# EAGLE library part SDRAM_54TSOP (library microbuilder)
64Mb SDRAM (4Mb x 16) Micron: MT48LC4M16A2P-7E:G TR - 133 MHz, 3V-3.6V, 0-70C - Digikey: 557-1089-1-ND MT48LC4M16A2P-75 IT:G TR - 133 MHz, 3V-3.6V, -40-85C - Digikey: 557-1087-1-ND ISSI (cheaper): IS42S16400F-7TL - 143 MHz, 3V-3.6V, 0-70C - Digikey: 706-1077-ND IS42S16400J-7TLI - 143 MHz, 3V-3.6V, -40-85C - Digikey: 706-1132-ND 256Mb SDRAM (16Mb x 16) MT48LC16M16A2TG-7E IT:D TR - 133MHz, 3V-3.6V, -40-85C - Digikey: 557-1064-1-ND
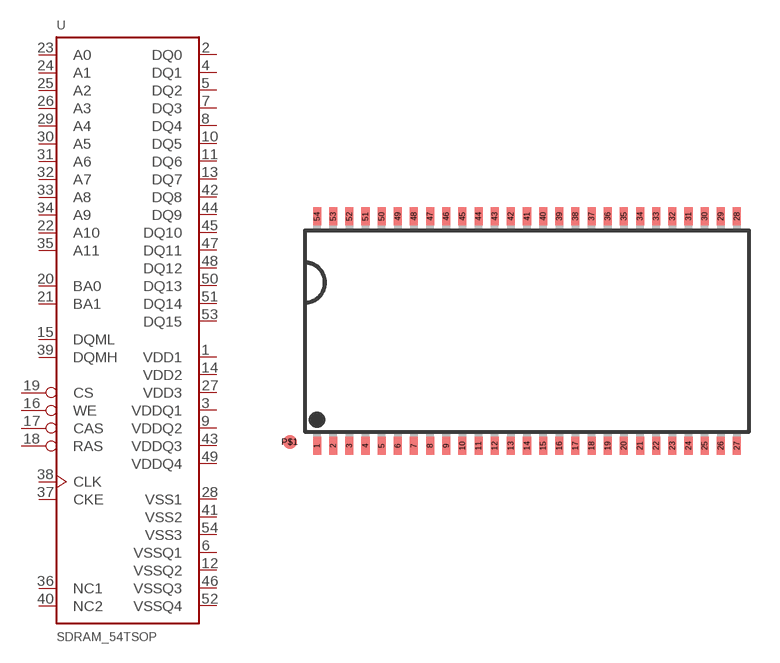
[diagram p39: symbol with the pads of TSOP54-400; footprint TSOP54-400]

Designator prefix U

## SDRAM_54TSOP  [TSOP54-400]
1  VDD1
2  DQ0
3  VDDQ1
4  DQ1
5  DQ2
6  VSSQ1
7  DQ3
8  DQ4
9  VDDQ2
10  DQ5
11  DQ6
12  VSSQ2
13  DQ7
14  VDD2
15  DQML
16  WE
17  CAS
18  RAS
19  CS
20  BA0
21  BA1
22  A10
23  A0
24  A1
25  A2
26  A3
27  VDD3
28  VSS1
29  A4
30  A5
31  A6
32  A7
33  A8
34  A9
35  A11
36  NC1
37  CKE
38  CLK
39  DQMH
40  NC2
41  VSS2
42  DQ8
43  VDDQ3
44  DQ9
45  DQ10
46  VSSQ3
47  DQ11
48  DQ12
49  VDDQ4
50  DQ13
51  DQ14
52  VSSQ4
53  DQ15
54  VSS3

## Footprint TSOP54-400 (pad centres in mm)
54-Pin Plastic TSOP (400 mil) Source: http://download.micron.com/pdf/datasheets/dram/sdram/256MSDRAM.pdf
smd 0.4 x 0.9: 1 -10.4,-5.68; 2 -9.6,-5.68; 3 -8.8,-5.68; 4 -8,-5.68; 5 -7.2,-5.68; 6 -6.4,-5.68; 7 -5.6,-5.68; 8 -4.8,-5.68; 9 -4,-5.68; 10 -3.2,-5.68; 11 -2.4,-5.68; 12 -1.6,-5.68; 13 -0.8,-5.68; 14 0,-5.68; 15 0.8,-5.68; 16 1.6,-5.68; 17 2.4,-5.68; 18 3.2,-5.68; 19 4,-5.68; 20 4.8,-5.68; 21 5.6,-5.68; 22 6.4,-5.68; 23 7.2,-5.68; 24 8,-5.68; 25 8.8,-5.68; 26 9.6,-5.68; 27 10.4,-5.68; 28 10.4,5.68; 29 9.6,5.68; 30 8.8,5.68; 31 8,5.68; 32 7.2,5.68; 33 6.4,5.68; 34 5.6,5.68; 35 4.8,5.68; 36 4,5.68; 37 3.2,5.68; 38 2.4,5.68; 39 1.6,5.68; 40 0.8,5.68; 41 0,5.68; 42 -0.8,5.68; 43 -1.6,5.68; 44 -2.4,5.68; 45 -3.2,5.68; 46 -4,5.68; 47 -4.8,5.68; 48 -5.6,5.68; 49 -6.4,5.68; 50 -7.2,5.68; 51 -8,5.68; 52 -8.8,5.68; 53 -9.6,5.68; 54 -10.4,5.68
smd 0.7 x 0.7: P$1 -11.75,-5.5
